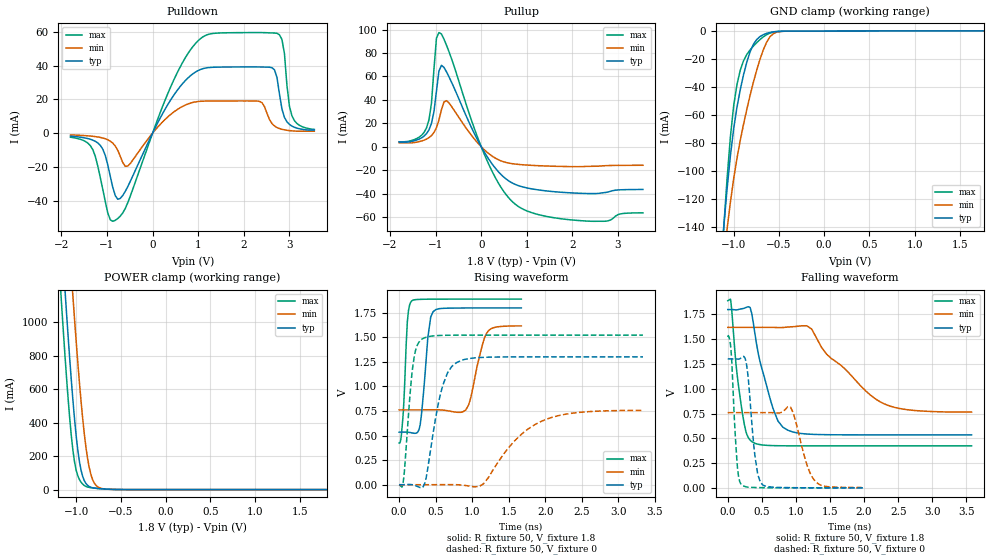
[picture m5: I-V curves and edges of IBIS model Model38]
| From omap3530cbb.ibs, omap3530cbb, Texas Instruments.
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| Model based on original model for BQOMAPPROGIOCSHYFBPB_7LM
|   Sub model MODE01_PD_ON_1P8
[model]   Model38
|[Input Load]   PD
|[Output Drive] DS01
|Voltage   1.8V
|Mode   I/O
Model_type   I/O
Polarity   Non-Inverting
Enable   Active-Low
Vinl =  0.63
Vinh =  1.17
Cref =  15.0000pF
Rref =  100.0000M
Vref =  0V
Vmeas =  0.9
C_comp   0.8864943p   0.7714798p   1.034566p
[Model Spec]
Vinl   0.63   0.567   0.6615
Vinh   1.17   1.053   1.2285
[Temperature Range]   25   125   -40
[Voltage Range]   1.8   1.62   1.89
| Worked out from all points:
|   slope of the pulldown table from 0 to 0.27 V, typ, clamps not added: 19.3 ohm
|   slope of the pullup table from 0 to 0.27 V, typ, clamps not added: 16.6 ohm
|   GND clamp passes 1 mA (typ) near -0.60 V on its own axis
|   POWER clamp passes 1 mA (typ) near -0.55 V on its own axis
|   rising waveform, R_fixture 50, V_fixture 1.8: 20-80 % time 87ps typ, 154ps min, 53.4ps max; typ from 0.535 V to 1.8 V
|   rising waveform, R_fixture 50, V_fixture 0: 20-80 % time 202ps typ, 557ps min, 101ps max; typ from 0 V to 1.3 V
|   falling waveform, R_fixture 50, V_fixture 1.8: 20-80 % time 271ps typ, 742ps min, 143ps max; typ from 1.8 V to 0.535 V
|   falling waveform, R_fixture 50, V_fixture 0: 20-80 % time 103ps typ, 185ps min, 68.7ps max; typ from 1.3 V to 0 V
[POWER_clamp]
-1.8V     7.429A     8.065A     7.064A
-1.182V   1.663A     2.35A      1.259A
-1.164V   1.508A     2.193A     1.106A
-1.127V   1.206A     1.883A     813.3mA
-1.073V   782.1mA    1.435A     426.3mA
-1.036V   530.7mA    1.15A      232.5mA
-981.8mV  234.7mA    756.3mA    81.79mA
-909.1mV  52.86mA    331.4mA    24.54mA
-872.7mV  25.66mA    185.5mA    15.5mA
-818.2mV  11.27mA    62mA       10.15mA
-709.1mV  4.611mA    6.166mA    4.556mA
1.8V      101uA      43.59uA    177.4uA
[Pulldown]
-1.8V     -1.789mA   -1.059mA   -2.429mA
-1.364V   -3.636mA   -1.733mA   -7.448mA
-1.145V   -7.295mA   -2.547mA   -26.48mA
-818.2mV  -36.98mA   -7.617mA   -51.58mA
-545.5mV  -31.67mA   -19.52mA   -41.22mA
654.5mV   29.22mA    15.79mA    41.66mA
1.527V    39.09mA    19.05mA    59.31mA
2.345V    39.14mA    18.78mA    59.5mA
2.618V    38.71mA    5.636mA    59.27mA
2.782V    23.04mA    2.689mA    58.16mA
3.055V    4.158mA    1.352mA    10.28mA
3.545V    1.801mA    1.153mA    2.203mA
[Pullup]
-1.8V     3.998mA    3.315mA    4.26mA
-1.2V     11.17mA    6.515mA    16.06mA
-1.091V   19.96mA    9.525mA    37.21mA
-1.036V   30.02mA    12.16mA    66.25mA
-981.8mV  47.48mA    16.29mA    92.64mA
-927.3mV  64.65mA    22.8mA     97.4mA
-872.7mV  69.46mA    31.49mA    96.17mA
-763.6mV  64.03mA    39.31mA    86.78mA
54.55mV   -3.696mA   -2.123mA   -5.186mA
709.1mV   -31.49mA   -14.6mA    -47.82mA
2.127V    -39.63mA   -17mA      -62.89mA
3.545V    -36.43mA   -15.79mA   -56.35mA
[GND_clamp]
-1.8V     -794.1mA   -670.5mA   -980.8mA
-1.109V   -139.6mA   -162.6mA   -140.1mA
-1.073V   -112.8mA   -141.5mA   -105.3mA
-1.036V   -89.25mA   -122.4mA   -75.78mA
-1V       -69.85mA   -105.6mA   -53.4mA
-963.6mV  -54.51mA   -90.99mA   -38.26mA
-890.9mV  -31.22mA   -66.62mA   -21.22mA
-818.2mV  -14.77mA   -45.88mA   -13.44mA
-709.1mV  -3.952mA   -20.19mA   -6.104mA
-600mV    -982.9uA   -4.198mA   -1.476mA
-490.9mV  -187.6uA   -374.7uA   -215.1uA
1.764V    101uA      43.71uA    177.3uA
[Ramp]
dV/dt_f  0.7758559/0.2720666n   0.525022/0.7524172n  0.9031477/0.1445672n
dV/dt_r  0.8003402/0.2017462n  0.4692705/0.5666845n  0.9361437/0.1018864n
R_load = 50
[Rising Waveform]
R_fixture = 50
V_fixture = 1.8
V_fixture_min = 1.62
V_fixture_max = 1.89
0s        534.8mV    761.4mV    423.9mV
56ps      535.4mV    761.4mV    731.9mV
112ps     534.6mV    761.4mV    1.657V
168ps     528.4mV    761.4mV    1.867V
288ps     610.5mV    761.4mV    1.886V
392ps     1.492V     762.2mV    1.888V
464ps     1.76V      762.6mV    1.888V
912ps     1.798V     761.3mV    1.888V
1.2ns     1.799V     1.544V     1.888V
1.672ns   1.799V     1.616V     1.888V
[Rising Waveform]
R_fixture = 50
V_fixture = 0
V_fixture_min = 0
V_fixture_max = 0
0s        241.7nV    156.4nV    521.6nV
64ps      646.2uV    2.79uV     74.73mV
160ps     1.606mV    3.124uV    1.013V
208ps     -5.714mV   152.5nV    1.31V
312ps     -31.99mV   -92.38uV   1.481V
576ps     952.7mV    867.4uV    1.519V
784ps     1.242V     291.7uV    1.522V
1.152ns   1.296V     7.839mV    1.522V
2.016ns   1.301V     666.7mV    1.522V
3.336ns   1.301V     755.7mV    1.522V
[Falling Waveform]
R_fixture = 50
V_fixture = 1.8
V_fixture_min = 1.62
V_fixture_max = 1.89
0s        1.799V     1.619V     1.888V
48ps      1.799V     1.619V     1.864V
128ps     1.796V     1.619V     1.201V
240ps     1.812V     1.619V     650.6mV
376ps     1.659V     1.619V     456.9mV
664ps     801mV      1.619V     426.3mV
880ps     582.1mV    1.623V     424.3mV
1.232ns   540.4mV    1.602V     423.9mV
2.272ns   534.8mV    854.8mV    423.9mV
3.576ns   534.8mV    764.7mV    423.9mV
[Falling Waveform]
R_fixture = 50
V_fixture = 0
V_fixture_min = 0
V_fixture_max = 0
0s        1.301V     759.1mV    1.522V
48ps      1.301V     759.1mV    1.388V
144ps     1.3V       759.1mV    190.5mV
200ps     1.315V     759.1mV    32.66mV
272ps     1.258V     759.1mV    10.05mV
400ps     315.6mV    759.1mV    3.516mV
480ps     53.24mV    759.1mV    2.095mV
920ps     2.151mV    815.2mV    60.33uV
1.336ns   247.5uV    36.67mV    1.802uV
2ns       10.84uV    3.313mV    450.9nV
